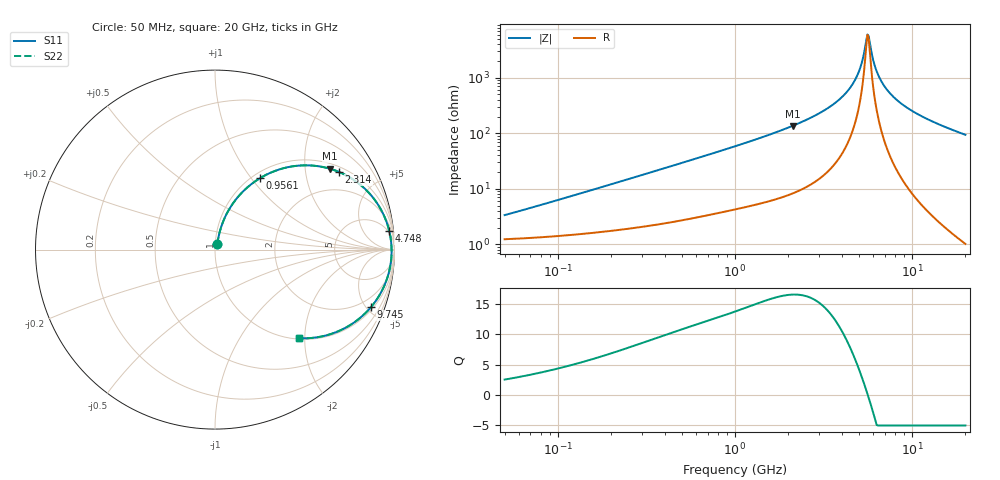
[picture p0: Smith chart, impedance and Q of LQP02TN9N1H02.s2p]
!Murata Part Number: LQP02TN9N1H02
!These Parameters are Measured in Series Mode Connection
!  o--[Z]--o
!Port1  Port2
!  o-------o
!Freq. Start=50[MHz] Stop=20[GHz], 401[Steps]
# Hz S RI R 50
!Freq.(Hz) S11(Real) S11(Imag) S21(Real) S21(Imag) S12(Real) S12(Imag) S22(Real) S22(Imag)
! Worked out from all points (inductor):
!   401 points, 50 MHz to 20 GHz, reference 50 ohm
!   read as one part in series: L = 9.83 nH near 61.67 MHz
!   highest Q = 16.5 at 2.115 GHz (marker M1), where L = 10.2 nH
!   self-resonance near 5.599 GHz
!   S11 on the Smith chart (normalised r, x): 50 MHz: 1.02, +0.06; 956.1 MHz: 1.08, +1.11; 2.314 GHz: 1.19, +3.07; 4.748 GHz: 4, +18; 9.745 GHz: 1.18, -5.32; 20 GHz: 1.02, -1.88
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5e7  0.0132 0.0305  0.9868 -0.0305  0.9868 -0.0305  0.0132 0.0305
1.364002e8  0.0216 0.0796  0.9784 -0.0796  0.9784 -0.0796  0.0216 0.0796
3.721004e8  0.065 0.1994  0.935 -0.1994  0.935 -0.1994  0.065 0.1994
9.560587e8  0.2521 0.3987  0.7479 -0.3987  0.7479 -0.3987  0.2521 0.3987
1e9  0.2683 0.408  0.7317 -0.408  0.7317 -0.408  0.2683 0.408
1.521052e9  0.4577 0.4672  0.5423 -0.4672  0.5423 -0.4672  0.4577 0.4672
2.114743e9  0.6412 0.4503  0.3588 -0.4503  0.3588 -0.4503  0.6412 0.4503
2.313601e9  0.6918 0.4324  0.3082 -0.4324  0.3082 -0.4324  0.6918 0.4324
2.728004e9  0.7797 0.3841  0.2203 -0.3841  0.2203 -0.3841  0.7797 0.3841
3.850025e9  0.9227 0.2267  0.0773 -0.2267  0.0773 -0.2267  0.9227 0.2267
4.34015e9  0.9542 0.1587  0.0458 -0.1587  0.0458 -0.1587  0.9542 0.1587
4.748272e9  0.9706 0.1049  0.0294 -0.1049  0.0294 -0.1049  0.9706 0.1049
5.117541e9  0.9794 0.0588  0.0206 -0.0588  0.0206 -0.0588  0.9794 0.0588
5.515528e9  0.9836 0.0121  0.0164 -0.0121  0.0164 -0.0121  0.9836 0.0121
5.598765e9  0.9839 0.00265  0.0161 -0.00265  0.0161 -0.00265  0.9839 0.00265
5.769027e9  0.9839 -0.0162  0.0161 0.0162  0.0161 0.0162  0.9839 -0.0162
6.125241e9  0.9818 -0.0538  0.0182 0.0538  0.0182 0.0538  0.9818 -0.0538
6.406762e9  0.9782 -0.0819  0.0218 0.0819  0.0218 0.0819  0.9782 -0.0819
7.442007e9  0.9545 -0.1736  0.0455 0.1736  0.0455 0.1736  0.9545 -0.1736
9.745021e9  0.868 -0.3218  0.132 0.3218  0.132 0.3218  0.868 -0.3218
1.396067e10  0.6833 -0.4564  0.3167 0.4564  0.3167 0.4564  0.6833 -0.4564
2e10  0.4691 -0.4937  0.5309 0.4937  0.5309 0.4937  0.4691 -0.4937
